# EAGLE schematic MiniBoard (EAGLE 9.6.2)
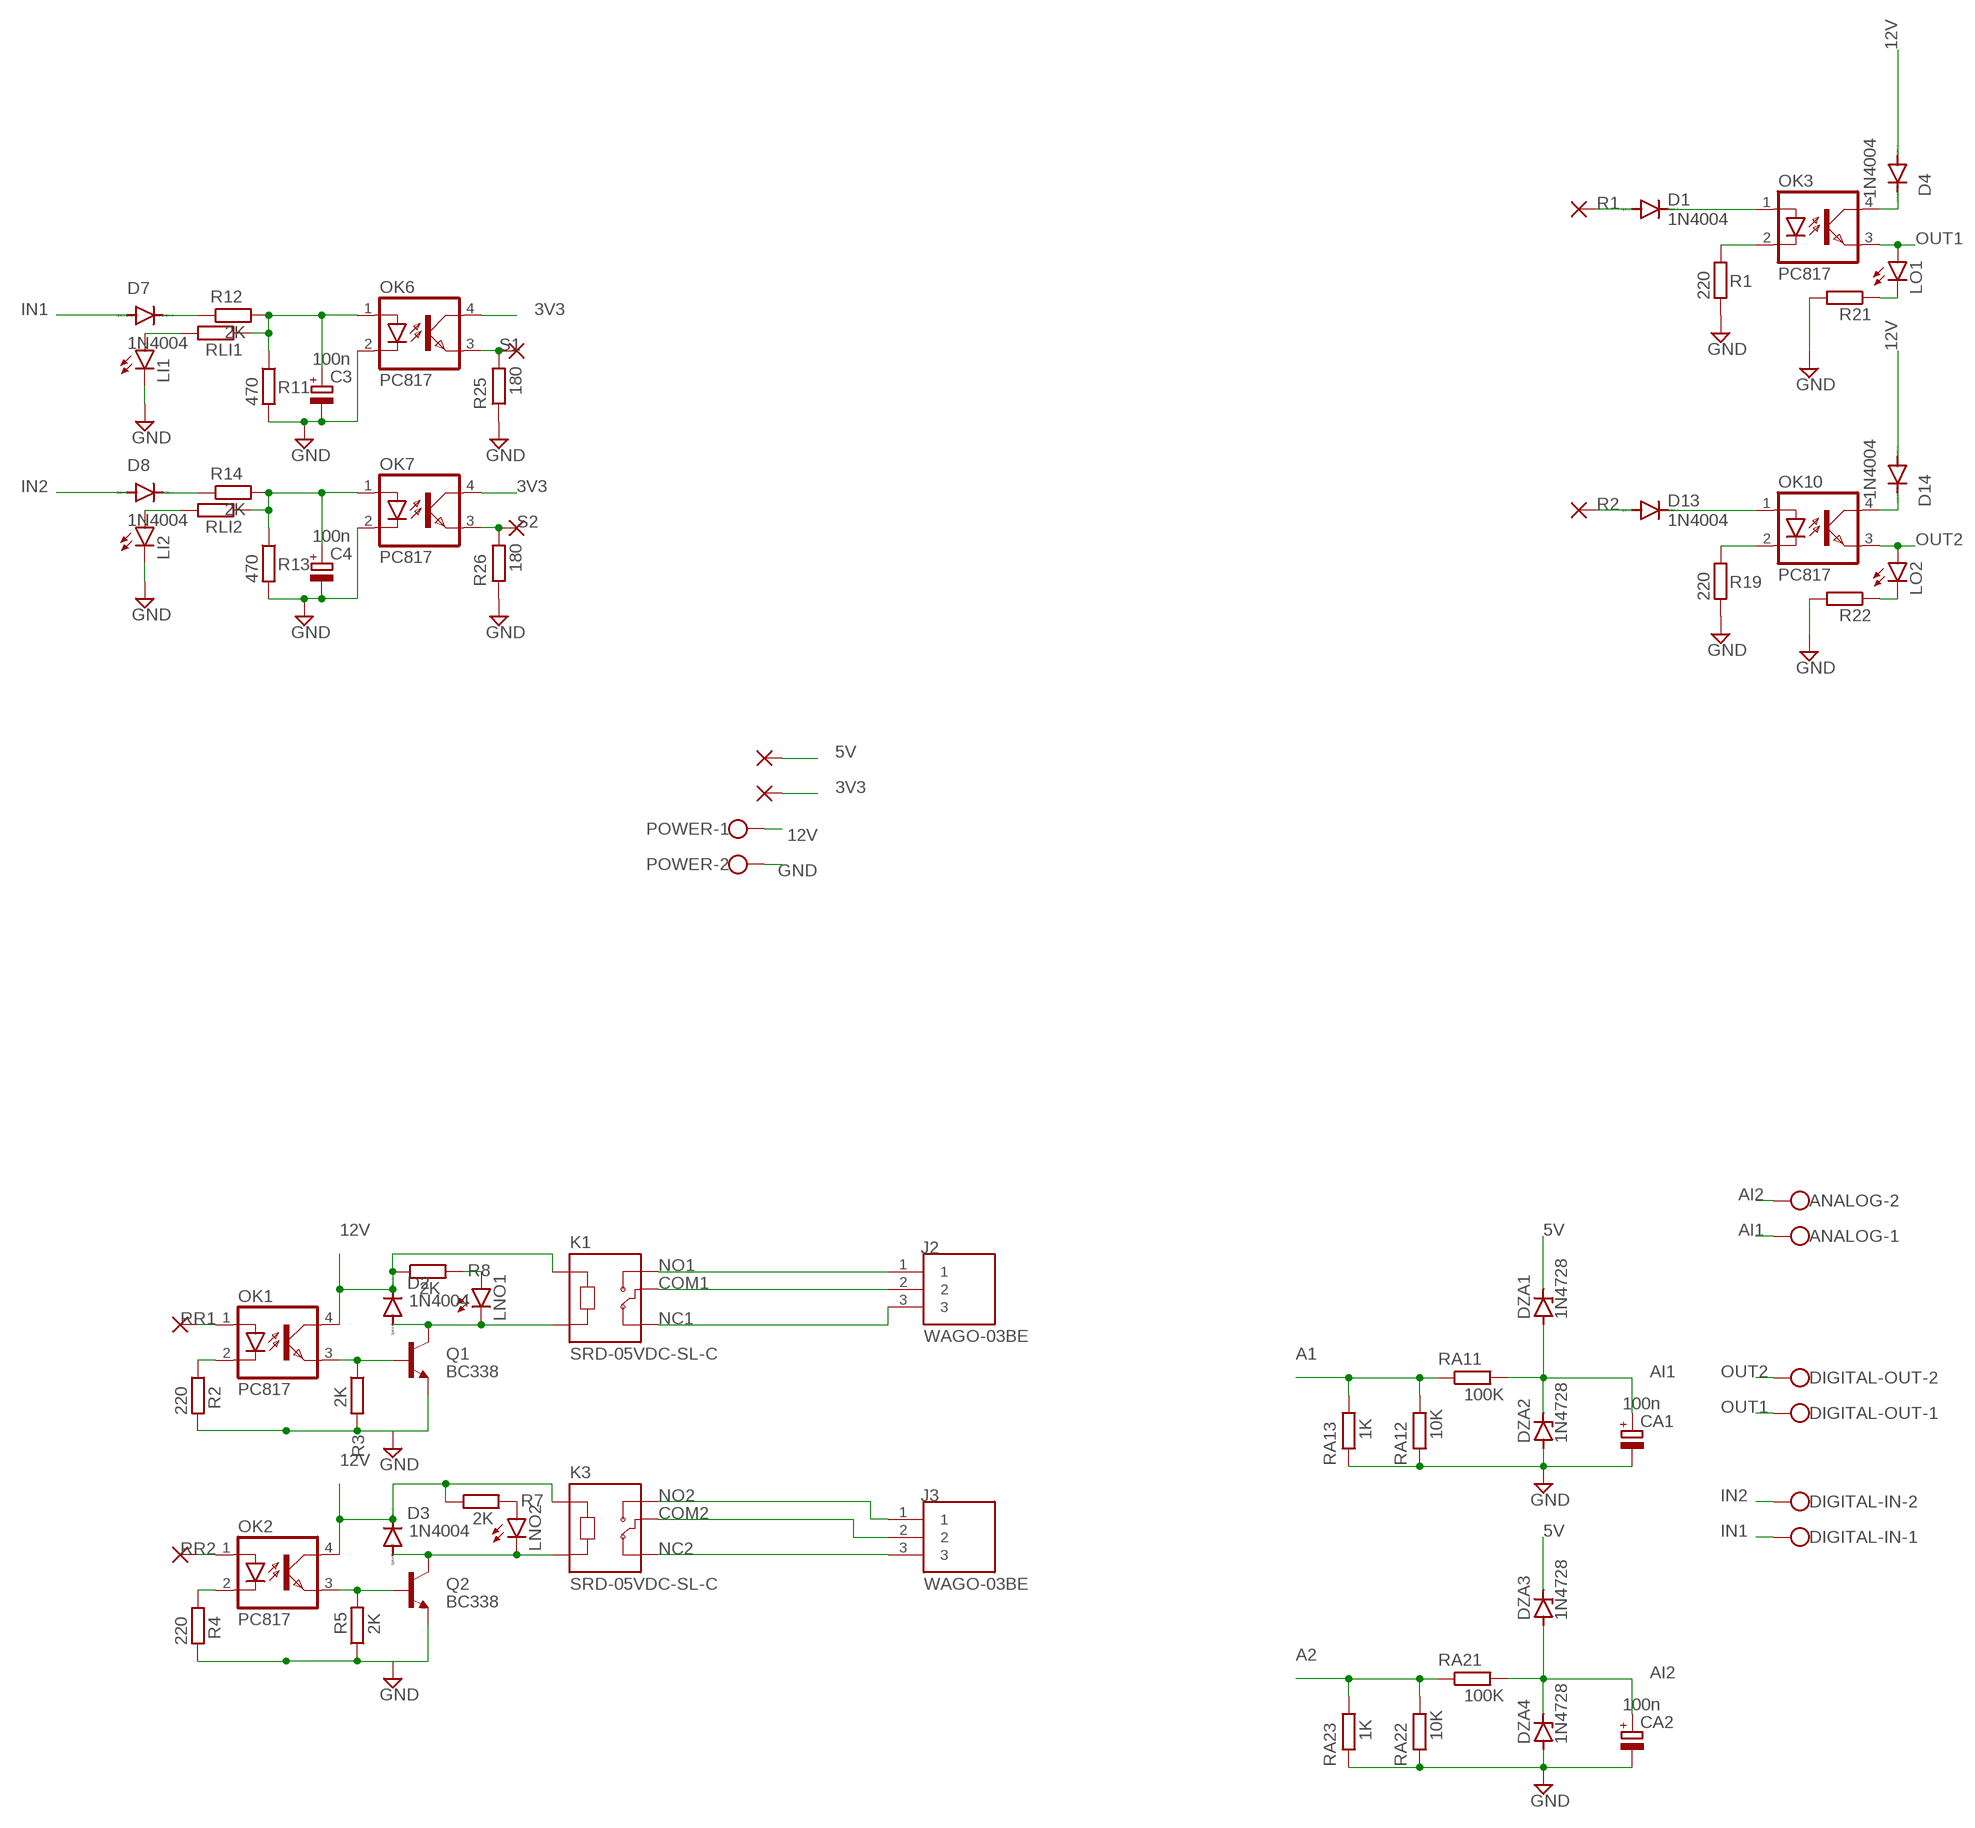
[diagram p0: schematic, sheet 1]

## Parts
ANALOG  W237-102  [W237-102]
C3  100n  CPOL-EUE5-6  [E5-6]
C4  100n  CPOL-EUE5-6  [E5-6]
CA1  100n  CPOL-EUE5-6  [E5-6]
CA2  100n  CPOL-EUE5-6  [E5-6]
D1  1N4004  [DO41-10]
D2  1N4004  [DO41-10]
D3  1N4004  [DO41-10]
D4  1N4004  [DO41-10]
D7  1N4004  [DO41-10]
D8  1N4004  [DO41-10]
D13  1N4004  [DO41-10]
D14  1N4004  [DO41-10]
DIGITAL-IN  W237-102  [W237-102]
DIGITAL-OUT  W237-102  [W237-102]
DZA1  1N4728  [DO41Z10]
DZA2  1N4728  [DO41Z10]
DZA3  1N4728  [DO41Z10]
DZA4  1N4728  [DO41Z10]
J2  WAGO-03BE  [CUI_TB006-508-03BE]
J3  WAGO-03BE  [CUI_TB006-508-03BE]
K1  SRD-05VDC-SL-C  [RELAY_SRD-05VDC-SL-C]
K3  SRD-05VDC-SL-C  [RELAY_SRD-05VDC-SL-C]
LI1  LED3MM  [LED3MM]
LI2  LED3MM  [LED3MM]
LNO1  LED3MM  [LED3MM]
LNO2  LED3MM  [LED3MM]
LO1  LED3MM  [LED3MM]
LO2  LED3MM  [LED3MM]
OK1  PC817  [DIL04]
OK2  PC817  [DIL04]
OK3  PC817  [DIL04]
OK6  PC817  [DIL04]
OK7  PC817  [DIL04]
OK10  PC817  [DIL04]
PAD1  WIREPAD1,6/0,9  [1,6/0,9]
PAD2  WIREPAD1,6/0,9  [1,6/0,9]
PAD3  WIREPAD1,6/0,9  [1,6/0,9]
PAD4  WIREPAD1,6/0,9  [1,6/0,9]
PAD5  WIREPAD1,6/0,9  [1,6/0,9]
PAD6  WIREPAD1,6/0,9  [1,6/0,9]
PAD79  WIREPAD1,6/0,9  [1,6/0,9]
PAD80  WIREPAD1,6/0,9  [1,6/0,9]
POWER  W237-102  [W237-102]
Q1  BC338  [TO92-EBC]
Q2  BC338  [TO92-EBC]
R1  220  R-EU_0309/12  [0309/12]
R2  220  R-EU_0309/12  [0309/12]
R3  2K  R-EU_0309/12  [0309/12]
R4  220  R-EU_0309/12  [0309/12]
R5  2K  R-EU_0309/12  [0309/12]
R7  2K  R-EU_0309/12  [0309/12]
R8  2K  R-EU_0309/12  [0309/12]
R11  470  R-EU_0309/12  [0309/12]
R12  2K  R-EU_0309/12  [0309/12]
R13  470  R-EU_0309/12  [0309/12]
R14  2K  R-EU_0309/12  [0309/12]
R19  220  R-EU_0309/12  [0309/12]
R21  R-EU_0309/12  [0309/12]
R22  R-EU_0309/12  [0309/12]
R25  180  R-EU_0309/12  [0309/12]
R26  180  R-EU_0309/12  [0309/12]
RA11  100K  R-EU_0309/12  [0309/12]
RA12  10K  R-EU_0309/12  [0309/12]
RA13  1K  R-EU_0309/12  [0309/12]
RA21  100K  R-EU_0309/12  [0309/12]
RA22  10K  R-EU_0309/12  [0309/12]
RA23  1K  R-EU_0309/12  [0309/12]
RLI1  R-EU_0309/12  [0309/12]
RLI2  R-EU_0309/12  [0309/12]

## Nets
3V3: OK6.4(COL) OK7.4(COL) PAD5.1(P)
5V: DZA1.C DZA3.C PAD6.1(P)
12V: D2.C D3.C D4.A D14.A K1.A1 K3.A1 OK1.4(COL) OK2.4(COL) POWER.1 R7.1 R8.1
A1: RA11.1 RA12.2 RA13.2
A2: RA21.1 RA22.2 RA23.2
AI1: ANALOG.1 CA1.+ DZA1.A DZA2.C RA11.2
AI2: ANALOG.2 CA2.+ DZA3.A DZA4.C RA21.2
COM1: J2.2 K1.COM
COM2: J3.2 K3.COM
GND: C3.- C4.- CA1.- CA2.- DZA2.A DZA4.A LI1.K(C) LI2.K(C) OK6.2(C) OK7.2(C) POWER.2 Q1.E Q2.E R1.2 R2.2 R3.2 R4.2 R5.1 R11.2 R13.2 R19.2 R21.2 R22.2 R25.1 R26.1 RA12.1 RA13.1 RA22.1 RA23.1
IN1: D7.A DIGITAL-IN.1
IN2: D8.A DIGITAL-IN.2
N$1: OK2.2(C) R4.1
N$2: OK1.2(C) R2.1
N$3: OK1.3(EMIT) Q1.B R3.1
N$4: D3.A K3.A2 LNO2.K(C) Q2.C
N$6: OK2.3(EMIT) Q2.B R5.2
N$7: LNO2.A R7.2
N$10: LNO1.A R8.2
N$11: D2.A K1.A2 LNO1.K(C) Q1.C
N$15: D1.C OK3.1(A)
N$16: OK3.2(C) R1.1
N$18: D4.C OK3.4(COL)
N$19: C3.+ OK6.1(A) R11.1 R12.2 RLI1.1
N$20: D7.C R12.1
N$21: C4.+ OK7.1(A) R13.1 R14.2 RLI2.1
N$22: D8.C R14.1
N$24: LI2.A RLI2.2
N$26: D13.C OK10.1(A)
N$27: OK10.2(C) R19.1
N$29: LI1.A RLI1.2
N$30: LO1.K(C) R21.1
N$31: LO2.K(C) R22.1
N$52: D14.C OK10.4(COL)
NC1: J2.3 K1.NC
NC2: J3.3 K3.NC
NO1: J2.1 K1.NO
NO2: J3.1 K3.NO
OUT1: DIGITAL-OUT.1 LO1.A OK3.3(EMIT)
OUT2: DIGITAL-OUT.2 LO2.A OK10.3(EMIT)
R1: D1.A PAD79.1(P)
R2: D13.A PAD80.1(P)
RR1: OK1.1(A) PAD4.1(P)
RR2: OK2.1(A) PAD3.1(P)
S1: OK6.3(EMIT) PAD1.1(P) R25.2
S2: OK7.3(EMIT) PAD2.1(P) R26.2

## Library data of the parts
ANALOG DIGITAL-IN DIGITAL-OUT POWER = con-wago-500:W237-102: WAGO SCREW CLAMP; MPN: 237-102; OC_FARNELL: unknown; OC_NEWARK: 70K9898
C3 C4 CA1 CA2 = rcl-ws:CPOL-EU: POLARIZED CAPACITOR, European symbol; SPICEPREFIX: C
D1-D4 D7 D8 D13 D14 = diode:1N4004: DIODE
DZA1-DZA4 = diode-ws:1N4728: Z DIODE
J2 J3 = TB006-508-03BE:WAGO-03BE: Check availability; AVAILABILITY: In Stock; CHECK_PRICES: https://www.snapeda.com/parts/TB006-508-03BE/Same+Sky/view-part/?ref=eda; DESCRIPTION: 2~24 Poles, Screw Type, Horizontal, 5.08 Pitch, 26~14 (AWG), Terminal Block Connector; MF: Same Sky; MP: TB006-508-03BE; PACKAGE: None; PRICE: None; SNAPEDA_LINK: https://www.snapeda.com/parts/TB006-508-03BE/Same+Sky/view-part/?ref=snap
K1 K3 = SRD-05VDC-SL-C:SRD-05VDC-SL-C: 5V Trigger Relay Module For Arduino And Raspberry Pi 5V Trigger Relay Module For Arduino And Raspberry Pi Check availability; AVAILABILITY: In Stock; CHECK_PRICES: https://www.snapeda.com/parts/SRD-05VDC-SL-C/Songle+Relay/view-part/?ref=eda; DESCRIPTION: 5V Trigger Relay Module For Arduino And Raspberry Pi 5V Trigger Relay Module For Arduino And Raspberry Pi; MF: Songle Relay; MP: SRD-05VDC-SL-C; PACKAGE: NON STANDARD-5 Songle Relay; PRICE: None; SNAPEDA_LINK: https://www.snapeda.com/parts/SRD-05VDC-SL-C/Songle+Relay/view-part/?ref=snap
LI1 LI2 LNO1 LNO2 LO1 LO2 = led_WS:LED: LED
OK1-OK3 OK6 OK7 OK10 = optocoupler:PC817: SHARP OPTO COUPLER; MPN: PC817X4J000F; OC_FARNELL: 9707727; OC_NEWARK: 97K7059
PAD1-PAD6 PAD79 PAD80 = wirepad-ws:WIREPAD: Wire PAD connect wire on PCB
Q1 Q2 = transistor-npn:BC338*: NPN Transistor
R1-R5 R7 R8 R11-R14 R19 R21 R22 R25 R26 RA11-RA13 RA21-RA23 RLI1 RLI2 = rcl-ws:R-EU_: RESISTOR, European symbol; SPICEPREFIX: R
